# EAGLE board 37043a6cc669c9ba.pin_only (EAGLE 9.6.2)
REV: C

Size 17.78 x 20.7 mm. Coordinates in mm from the lower left corner, seen from the top.
Outline: 17.78,18.16 17.78,2.54 arc-90 15.24,0 2.54,0 arc-90 0,2.54 0,18.16 arc-90 2.54,20.7 15.24,20.7 arc-90 17.78,18.16
Copper layers (1*16): Top 0.035mm / dielectric 1.5mm / Bottom 0.035mm
Design rules "adafruit 6-6 *": minimum track width 6mil, minimum drill 15.5mil, track to track 6mil, track to pad 6mil, pad to pad 6mil, via to via 6mil, smd to smd 6mil, copper to edge 10mil, drill to drill 8mil, minimum pad ring 10mil, minimum via ring 8mil, stop-mask expansion 2mil, vias tented up to drill 20mil, thermal gap 10mil
Net classes: 1 power: width 0.305 mm; 2 gnd: width 0.254 mm

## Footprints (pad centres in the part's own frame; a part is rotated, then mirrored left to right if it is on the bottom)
0805-NO = smd 1.24 x 1.5: 1 -0.95,0; 2 0.95,0
0603-NO = smd 1.075 x 1: 1 -0.85,0; 2 0.85,0
_0402NO = smd 0.6 x 0.6: 1 -0.508,0; 2 0.508,0
JST_SH4_SKINNY = smd 0.5 x 1.55: 1 -1.5,2.514; 2 -0.5,2.514; 3 0.5,2.514; 4 1.5,2.514 | smd 1.2 x 1.8: MT1 -2.8,-1.386; MT2 2.8,-1.386
SOD-323_MINI = smd 0.9 x 0.8: A 1.07,0; C -1.07,0
QFN56_7MM_REDUCEDEPAD = smd 0.875 x 0.2: 1 -3.45,2.6; 2 -3.45,2.2; 3 -3.45,1.8; 4 -3.45,1.4; 5 -3.45,1; 6 -3.45,0.6; 7 -3.45,0.2; 8 -3.45,-0.2; 9 -3.45,-0.6; 10 -3.45,-1; 11 -3.45,-1.4; 12 -3.45,-1.8; 13 -3.45,-2.2; 14 -3.45,-2.6; 29 3.45,-2.6; 30 3.45,-2.2; 31 3.45,-1.8; 32 3.45,-1.4; 33 3.45,-1; 34 3.45,-0.6; 35 3.45,-0.2; 36 3.45,0.2; 37 3.45,0.6; 38 3.45,1; 39 3.45,1.4; 40 3.45,1.8; 41 3.45,2.2; 42 3.45,2.6 | smd 0.2 x 0.875: 15 -2.6,-3.45; 16 -2.2,-3.45; 17 -1.8,-3.45; 18 -1.4,-3.45; 19 -1,-3.45; 20 -0.6,-3.45; 21 -0.2,-3.45; 22 0.2,-3.45; 23 0.6,-3.45; 24 1,-3.45; 25 1.4,-3.45; 26 1.8,-3.45; 27 2.2,-3.45; 28 2.6,-3.45; 43 2.6,3.45; 44 2.2,3.45; 45 1.8,3.45; 46 1.4,3.45; 47 1,3.45; 48 0.6,3.45; 49 0.2,3.45; 50 -0.2,3.45; 51 -0.6,3.45; 52 -1,3.45; 53 -1.4,3.45; 54 -1.8,3.45; 55 -2.2,3.45; 56 -2.6,3.45 | smd 3.2 x 3.2: P$1 0,0
1X07_CASTEL = drill 1 pad 1.778: 1 -7.62,0; 2 -5.08,0; 3 -2.54,0; 4 0,0; 5 2.54,0; 6 5.08,0; 7 7.62,0 | drill 1 pad 1.778 long: 1C -7.62,-1.27; 2C -5.08,-1.27; 3C -2.54,-1.27; 4C 0,-1.27; 5C 2.54,-1.27; 6C 5.08,-1.27; 7C 7.62,-1.27
SJ_2S-NO = smd 0.635 x 1.27: 1 -0.45,0; 2 0.45,0
SK6805_1515 = smd 0.5 x 0.5: 1 -0.5,-0.45; 2 0.5,-0.45; 3 0.5,0.45; 4 -0.5,0.45
BTN_KMR2_4.6X2.8 = smd 0.9 x 0.9: A 2.05,0.8; A' -2.05,0.8; B 2.05,-0.8; B' -2.05,-0.8
TESTPOINT_ROUND_1.5MM_NO = smd 1.5 x 1.5: P$1 0,0
SOT23-5 = smd 0.55 x 1.2: 1 -0.95,-1.3; 2 0,-1.3; 3 0.95,-1.3; 4 0.95,1.3; 5 -0.95,1.3
USON8_4X4 = smd 0.6 x 0.4: 1 -1.85,1.2; 2 -1.85,0.4; 3 -1.85,-0.4; 4 -1.85,-1.2; 5 1.85,-1.2; 6 1.85,-0.4; 7 1.85,0.4; 8 1.85,1.2 | smd 2 x 3: PAD 0,0
FIDUCIAL_1MM = smd 1 x 1: 1 0,0
USB_C_CUSB31-CFM2AX-01-X = smd 0.575 x 1.15: A1B12 -3.2,3.545; A4B9 -2.4,3.545; B1A12 3.2,3.545; B4A9 2.4,3.545 | smd 0.275 x 1.15: A5 -1.25,3.545; A6 -0.25,3.545; A7 0.25,3.545; A8 1.25,3.545; B5 1.75,3.545; B6 0.75,3.545; B7 -0.75,3.545; B8 -1.75,3.545 | drill 0.6 pad 1 long: M1 -4.32,2.97; M2 4.32,2.97; M3 -4.32,-1.21; M4 4.32,-1.21 | hole 0.65: 2.89,2.47; -2.89,2.47
CRYSTAL_2.5X2 = smd 0.9 x 0.75: 1 -0.825,-0.625; 2 0.825,-0.625; 3 0.825,0.625; 4 -0.825,0.625

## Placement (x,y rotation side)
C1  10uF  [0805-NO]  13.28,11.95 90 top
C2  1uF  [0603-NO]  13.61,12.2 180 bottom
C7  0.1uF  [_0402NO]  6.1,1.88 180 bottom
C8  10uF  [0805-NO]  8.71,7.05 0 top
C9  0.1uF  [_0402NO]  13.68,10.38 90 bottom
C10  1uF  [0603-NO]  4.29,2.23 270 bottom
C11  0.1uF  [_0402NO]  6.77,11.86 270 bottom
C12  1uF  [0603-NO]  5.37,12.23 90 bottom
C13  0.1uF  [_0402NO]  7.18,13.3 0 bottom
C14  0.1uF  [_0402NO]  3.95,11.75 90 bottom
C16  0.1uF  [_0402NO]  11.49,8.83 90 top
C17  0.1uF  [_0402NO]  14,4.78 270 bottom
C19  22pF  [_0402NO]  12.89,2.29 0 bottom
C20  22pF  [_0402NO]  12.89,0.95 0 bottom
CONN1  STEMMA_I2C_QTSKINNY  [JST_SH4_SKINNY]  7.01,2.39 0 top
D1  NSR0320  [SOD-323_MINI]  11.72,11.89 90 top
D2  NSR0320  [SOD-323_MINI]  7.26,19.23 180 bottom
IC2  RP2040_QFN56  [QFN56_7MM_REDUCEDEPAD]  9.14,7 0 bottom
JP1  [1X07_CASTEL]  1.27,10.35 270 top
JP2  [SJ_2S-NO]  13.21,17.08 0 bottom
JP3  [1X07_CASTEL]  16.51,10.35 90 top
LED1  WS2812B_SK6805_1515  [SK6805_1515]  13.35,6.4 90 top
R3  10K  [_0402NO]  5.85,16.88 270 bottom
R6  1K  [_0402NO]  8.7,1.52 90 bottom
R9  10K  [_0402NO]  11.49,6.71 270 top
R12  5.1K  [_0402NO]  5.55,12.92 0 top
R13  5.1K  [_0402NO]  10.43,12.61 90 top
R14  27  [_0402NO]  9.31,12.61 270 top
R15  27  [_0402NO]  7.28,12.48 270 top
R16  1K  [_0402NO]  10.13,19.33 0 bottom
SW1  KMR2  [BTN_KMR2_4.6X2.8]  12.51,2.79 90 top
SW2  KMR2  [BTN_KMR2_4.6X2.8]  5.16,9.4 90 top
TP3  [TESTPOINT_ROUND_1.5MM_NO]  15.34,1.02 0 bottom
TP4  [TESTPOINT_ROUND_1.5MM_NO]  3.34,17.31 0 bottom
U1  AP2112K-3.3  [SOT23-5]  8.84,9.68 90 top
U5  8MB QSPI Flash  [USON8_4X4]  8.57,15.94 270 bottom
U$1  [QTPICO_BOT]  17.78,0.06 0 bottom
U$2  [QTPICO_TOP]  0,0 0 top
U$6  FIDUCIAL_1MM  [FIDUCIAL_1MM]  2.49,19.63 0 bottom
U$8  FIDUCIAL_1MM  [FIDUCIAL_1MM]  8.89,17.78 0 top
X2  USB Type C  [USB_C_CUSB31-CFM2AX-01-X]  8.89,17.92 180 top
Y1  12MHZ  [CRYSTAL_2.5X2]  10.5,1.61 0 bottom

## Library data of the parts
C1 C2 C7-C14 C16 C17 C19 C20 CONN1 D1 D2 JP1 JP3 LED1 R3 R6 R9 R12-R16 SW1 SW2 TP3 TP4 U5 X2 Y1 = microbuilder
IC2 = adafruit_micro
JP2 = SparkFun
U1 = adafruit_power
U$1 U$2 = itsy_silks
U$6 U$8 = microbuilder; BOM: EXCLUDE

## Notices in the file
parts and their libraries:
microbuilder: This work is placed in the public domain, and may be freely used for commercial and non-commercial work with the following conditions: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
SparkFun: Licensing: CC v3.0 Share-Alike You are welcome to use this library for commercial purposes.
